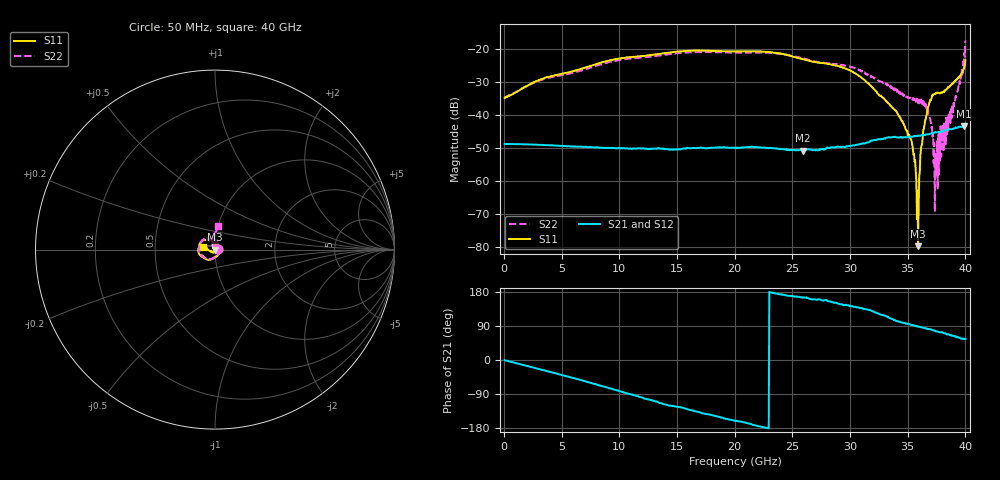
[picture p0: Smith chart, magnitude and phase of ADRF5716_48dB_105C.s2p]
! Device: ADRF5716
! Description: 30GHz 2-Bit Digital Attenuator
! Frequency: 100 MHz – 30 GHz
! Ports:
! ATTIN  = Port 1
! ATTOUT = Port 2
! State: 48 dB Attenuation selected
! Supply Voltage:
! VDD  =  +3.30 Volts
! VSS  =  -3.30 Volts
! Control Voltages:
! D5 = 3.3V, D6 = 3.3V
! Temperature = +105 C
! Data: Data was collected using a calibrated network analyzer.
!  The reference plane is the package pins of ADRF5716 switch.
! Note: Analog Devices supplies this data as a sample of measured data for this product.
!  Your particular data for this product may vary.
!  Analog Devices reserves the right to change this data at anytime
# HZ S DB R 50
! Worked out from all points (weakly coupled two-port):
!   800 points, 50 MHz to 40 GHz, reference 50 ohm
!   highest |S21| = -43.46 dB at 39.85 GHz (marker M1); lowest = -50.8 dB at 25.9 GHz (marker M2)
!   lowest |S11| = -79.8 dB at 35.9 GHz (marker M3), VSWR 1.00, Z = 50 + j0.0103 ohm
!   |S11| at or under -10 dB: start of sweep to end of sweep
!   |S22| runs from -69.3 to -17.5 dB; largest |S21 - S12| = 0
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5e7  -34.90 4.6  -48.81 -0.4  -48.81 -0.4  -35.00 4.6
6.75e9  -26.01 -101.1  -49.66 -53.6  -49.66 -53.6  -26.58 -100.7
1.34e10  -21.59 -151.0  -50.17 -112.2  -50.17 -112.2  -22.08 -153.5
2.005e10  -20.84 168.2  -49.98 -160.7  -49.98 -160.7  -21.15 163.0
2.59e10  -23.16 130.4  -50.81 164.7  -50.81 164.7  -22.95 120.8
2.67e10  -23.87 127.6  -50.61 160.2  -50.61 160.2  -23.75 115.9
3.015e10  -26.86 102.0  -49.38 141.7  -49.38 141.7  -25.57 89.0
3.335e10  -36.64 88.6  -46.72 111.9  -46.72 111.9  -31.27 58.7
3.525e10  -47.36 101.9  -46.52 93.3  -46.52 93.3  -34.78 41.1
3.555e10  -51.89 100.2  -46.35 90.6  -46.35 90.6  -35.16 37.1
3.575e10  -59.84 100.0  -46.45 90.1  -46.45 90.1  -35.13 35.8
3.59e10  -79.75 92.5  -46.27 88.5  -46.27 88.5  -36.44 36.2
3.6e10  -58.82 -77.8  -46.33 87.6  -46.33 87.6  -36.53 33.4
3.625e10  -48.87 -91.5  -46.13 86.0  -46.13 86.0  -35.79 23.4
3.655e10  -41.23 -98.4  -45.96 84.2  -45.96 84.2  -36.69 12.1
3.7e10  -35.62 -120.5  -45.70 80.4  -45.70 80.4  -42.17 -36.6
3.73e10  -33.75 -136.9  -45.43 77.2  -45.43 77.2  -48.61 -75.2
3.75e10  -33.47 -144.5  -45.33 75.4  -45.33 75.4  -58.32 -133.1
3.785e10  -33.40 -150.8  -45.30 73.1  -45.30 73.1  -43.50 112.0
3.945e10  -28.70 -177.4  -43.57 58.8  -43.57 58.8  -31.70 123.9
3.985e10  -26.34 169.7  -43.46 55.3  -43.46 55.3  -25.46 102.7
4e10  -23.49 168.1  -43.52 55.5  -43.52 55.5  -17.51 82.3
